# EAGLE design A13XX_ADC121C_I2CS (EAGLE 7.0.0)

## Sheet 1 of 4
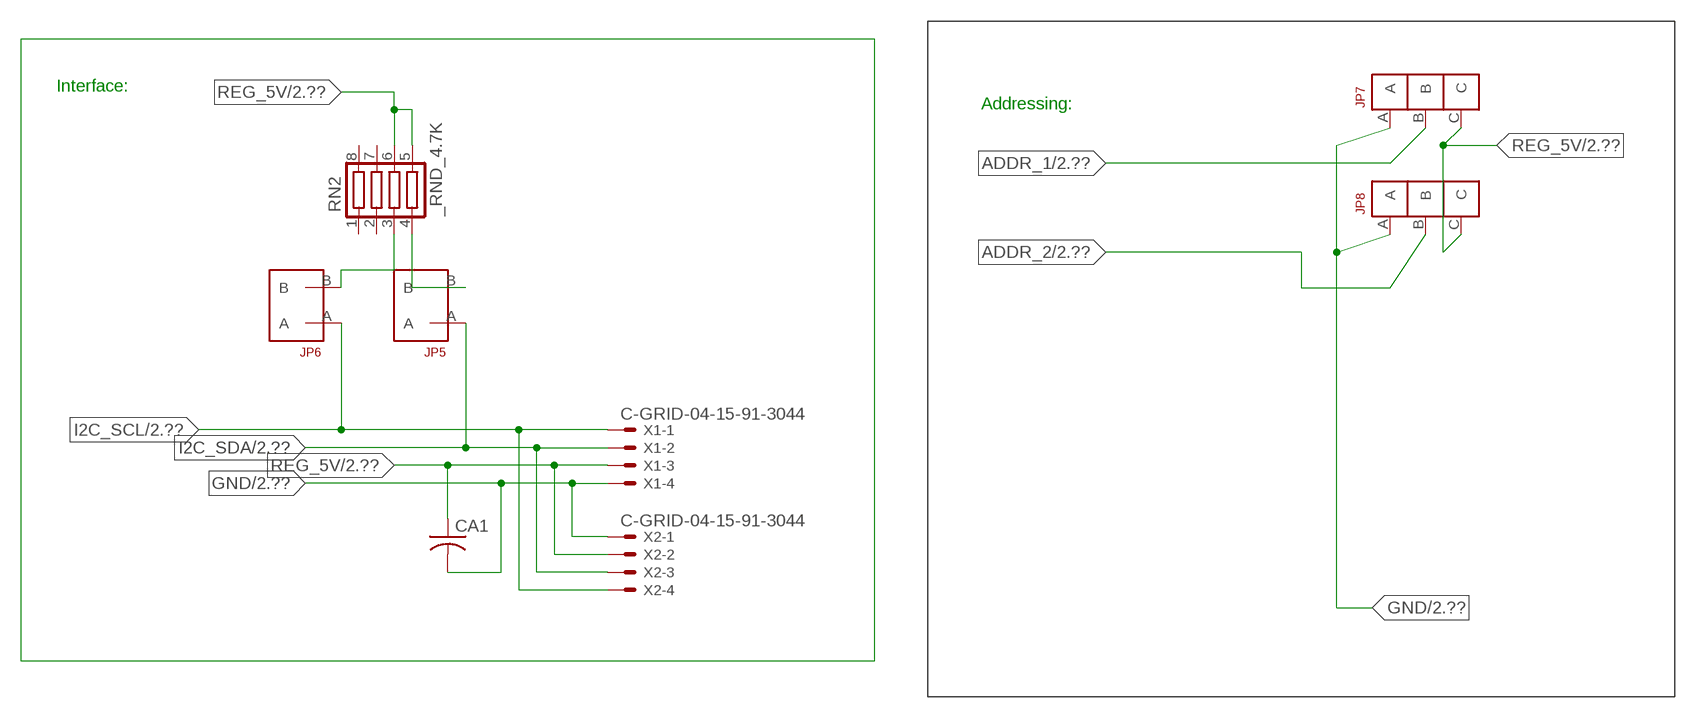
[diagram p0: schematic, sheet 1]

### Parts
CA1  CC1206KRX7R9BB104  [.1UF]
JP5  JUMPER_1X2_2MM  [JUMPER_1X2_2MM]
JP6  JUMPER_1X2_2MM  [JUMPER_1X2_2MM]
JP7  JUMPER_1X3_2MM  [JUMPER_1X3_2MM]
JP8  JUMPER_1X3_2MM  [JUMPER_1X3_2MM]
RN2  _RND_4.7K  [RND]
X1  C-GRID-04-15-91-3044  [15-91-04]
X2  C-GRID-04-15-91-3044  [15-91-04]

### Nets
ADDR_1: JP7.B ; also sheet 2
ADDR_2: JP8.B ; also sheet 2
GND: CA1.2 JP7.A JP8.A X1.4 X2.1 ; also sheet 2,3,4
I2C_SCL: JP6.A X1.1 X2.4 ; also sheet 2
I2C_SDA: JP5.A X1.2 X2.3 ; also sheet 2
N$1: JP6.B RN2.3
N$2: JP5.B RN2.4
REG_5V: CA1.1 JP7.C JP8.C RN2.5 RN2.6 X1.3 X2.2 ; also sheet 2,3,4
Unconnected: RN2.1 RN2.2 RN2.7 RN2.8

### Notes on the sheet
- Interface:
- Addressing:

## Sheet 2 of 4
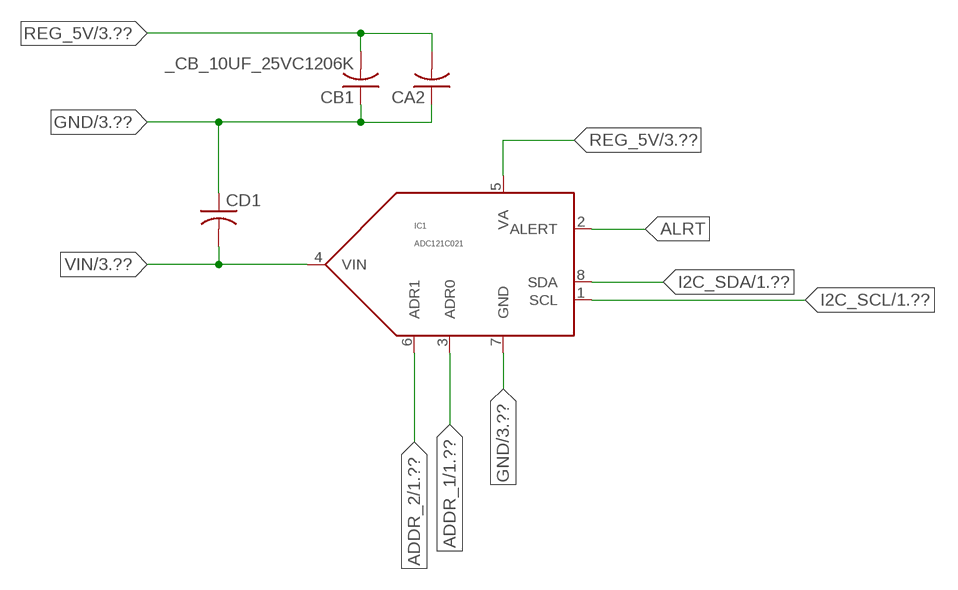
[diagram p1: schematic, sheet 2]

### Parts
CA2  _CA_.10UF_50VC1206K  [_CA_.1UF_50V]
CB1  _CB_10UF_25VC1206K  [_CB_10UF_25V]
CD1  _CD_10NF_50VC1206K  [_CD_10NF_50V]
IC1  ADC121C021  [MSOP08]

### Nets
ADDR_1: IC1.3(ADR0) ; also sheet 1
ADDR_2: IC1.6(ADR1) ; also sheet 1
ALRT: IC1.2(ALERT)
GND: CA2.1 CB1.1 CD1.1 IC1.7(GND) ; also sheet 1,3,4
I2C_SCL: IC1.1(SCL) ; also sheet 1
I2C_SDA: IC1.8(SDA) ; also sheet 1
REG_5V: CA2.2 CB1.2 IC1.5(VA) ; also sheet 1,3,4
VIN: CD1.2 IC1.4(VIN) ; also sheet 3

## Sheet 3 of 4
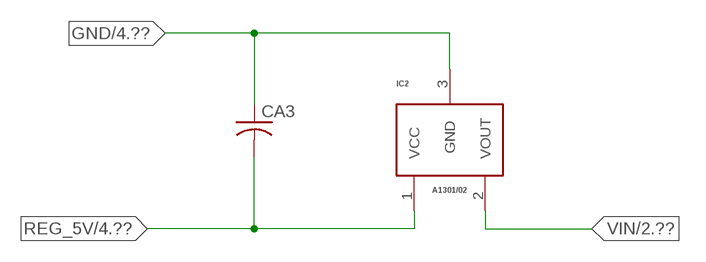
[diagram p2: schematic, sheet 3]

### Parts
CA3  _CA_.10UF_50VC1206K  [_CA_.1UF_50V]
IC2  A1301/02  [SOT23]

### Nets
GND: CA3.1 IC2.3(GND) ; also sheet 1,2,4
REG_5V: CA3.2 IC2.1(VCC) ; also sheet 1,2,4
VIN: IC2.2(VOUT) ; also sheet 2

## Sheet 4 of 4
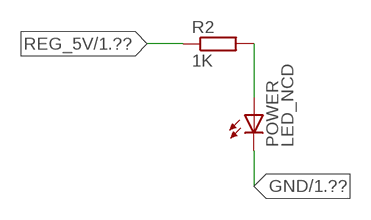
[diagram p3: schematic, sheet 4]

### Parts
POWER  LED_NCD  [CHIPLED_0603]
R2  1K  RESISTOR_SMT-0402  [R402]

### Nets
GND: POWER.C ; also sheet 1,2,3
N$13: POWER.A R2.2
REG_5V: R2.1 ; also sheet 1,2,3

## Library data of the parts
CA1 = NCD_ULTIMATE_LIBRARY:CC1206KRX7R9BB104: Capacitor CA .1uF 50V SMT C1206K CC1206KRX7R9BB104
CA2 CA3 = NCD_ULTIMATE_LIBRARY:_CA_.10UF_50V: Capacitor .1uF SMT
CB1 = NCD_ULTIMATE_LIBRARY:_CB_10UF_25V: Capacitor 10uF SMT
CD1 = NCD_ULTIMATE_LIBRARY:_CD_10NF_50V: Capacitor 10nF SMT
IC1 = NCD_ULTIMATE_bhaskar:ADC121C021: Digikey ADC121C021CIMM/NOPBCT-ND/ADC121C021CIMM/NOPB
IC2 = NCD_ULTIMATE_bhaskar:A1301/02: Digikey 620-1019-2-ND/A1301KLHLT-T 620-1021-2-ND/A1302KLHLT-T
JP5 JP6 = NCD_ULTIMATE_CONNECTORS:JUMPER_1X2_2MM
JP7 JP8 = NCD_ULTIMATE_CONNECTORS:JUMPER_1X3_2MM
POWER = NCD_ULTIMATE_LIBRARY:LED_NCD: LED Digikey 754-1132-2-ND/APT2012SRCPRV
R2 = NCD_ULTIMATE_LIBRARY:RESISTOR_SMT: NCD Resistor
RN2 = NCD_ULTIMATE_LIBRARY:_RND_4.7K: Resistor Array RND SMT 4.7K x 4 Single Resistor Source: http://www.ctscorp.com/components/Datasheets/CTSChipArrayDs.pdf Digikey 742C083472JPTR-ND/742C083472JP; OC_FARNELL: unknown; OC_NEWARK: unknown
X1 X2 = NCD_ULTIMATE_CONNECTORS:C-GRID-04: CONNECTOR 4-Pos I2C wire to board 2.54 mm (0.100") pitch header Digikey WM1342-ND/0015912045; OC_FARNELL: unknown; OC_NEWARK: unknown

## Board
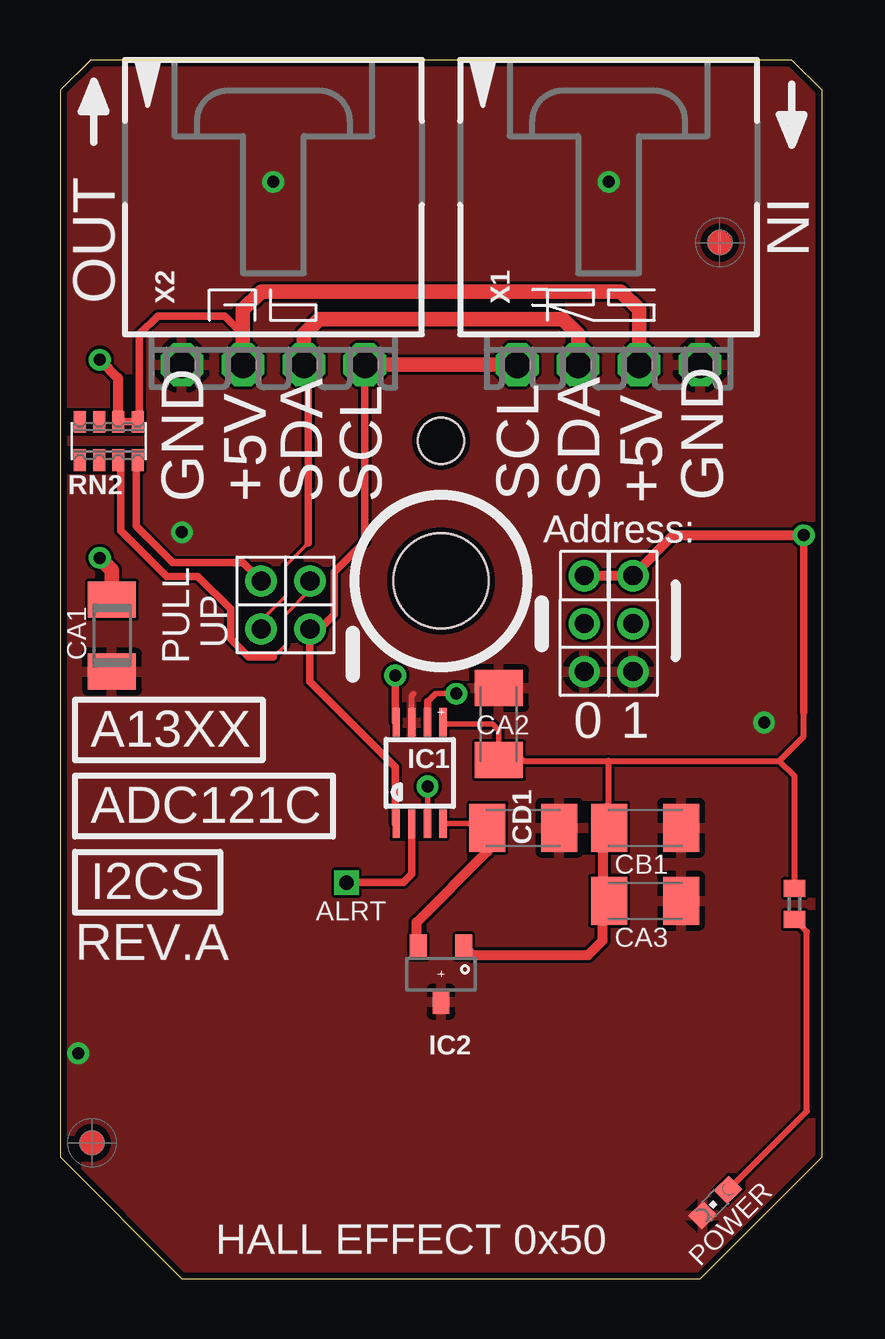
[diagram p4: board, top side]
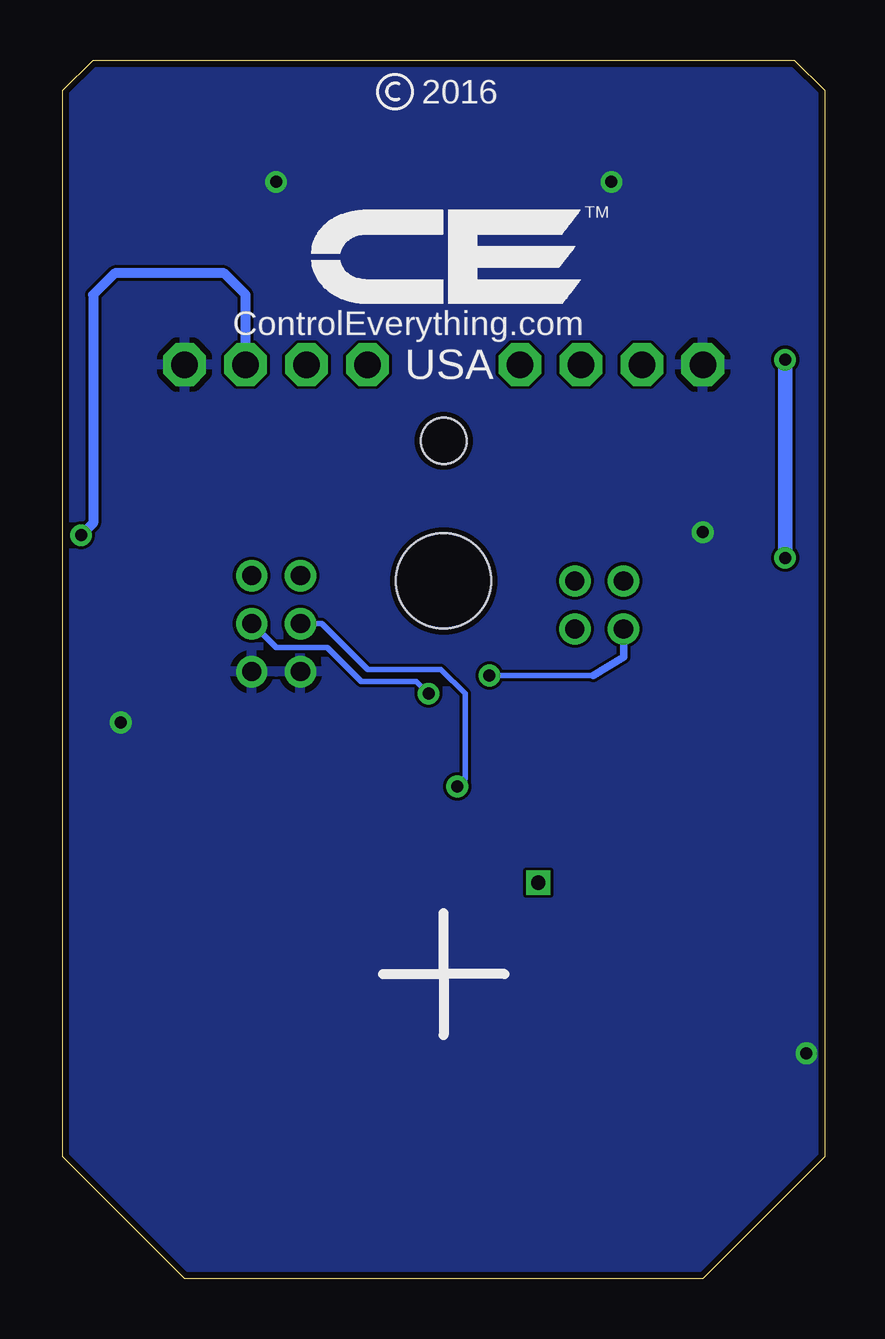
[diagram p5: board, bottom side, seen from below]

Size 31.75 x 50.8 mm. Coordinates in mm from the lower left corner, seen from the top.
Outline: 31.75,5.08 31.75,49.53 30.48,50.8 1.27,50.8 0,49.53 0,5.08 5.08,0 26.67,0 31.75,5.08
Outline: 31.75,5.08 31.75,49.53 30.48,50.8 1.27,50.8 0,49.53 0,5.08 5.08,0 26.67,0 31.75,5.08
Copper layers (1*16): Top 0.035mm / dielectric 1.5mm / Bottom 0.035mm
Design rules "default": minimum track width 5mil, minimum drill 24mil, track to track 5mil, track to pad 5mil, pad to pad 5mil, via to via 5mil, smd to smd 5mil, copper to edge 10mil, drill to drill 8mil, minimum pad ring 10mil, minimum via ring 8mil, stop-mask expansion 2mil, vias tented up to drill 0mil, thermal gap 10mil
Holes 3.96 mm at 15.88,29.08
Holes 1.91 mm at 15.88,34.92

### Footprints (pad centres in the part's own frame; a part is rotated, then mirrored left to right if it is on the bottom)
.1UF = smd 1.5 x 2: 1 -1.5,0; 2 1.5,0
_CA_.1UF_50V = smd 1.5 x 2: 1 -1.5,0; 2 1.5,0
_CB_10UF_25V = smd 1.5 x 2: 1 -1.5,0; 2 1.5,0
_CD_10NF_50V = smd 1.5 x 2: 1 -1.5,0; 2 1.5,0
MSOP08 = smd 0.3 x 1.2: 1 -0.976,-2.113; 2 -0.326,-2.113; 3 0.324,-2.113; 4 0.974,-2.113; 5 0.974,2.112; 6 0.324,2.112; 7 -0.326,2.112; 8 -0.976,2.112
SOT23 = smd 0.7 x 1: 1 -0.95,-1.15; 2 0.95,-1.15; 3 0,1.15
JUMPER_1X2_2MM = drill 0.8: A 0,2; B 0,0
JUMPER_1X3_2MM = drill 0.8: A 0,2; B 0,0; C 0,-2
CHIPLED_0603 = smd 0.8 x 0.876: A 0,-0.75; C 0,0.75
R402 = smd 0.7 x 0.9: 1 -0.65,0; 2 0.65,0
RND = smd 0.5 x 0.9: 1 -1.2,-0.8; 2 -0.4,-0.8; 3 0.4,-0.8; 4 1.2,-0.8; 5 1.2,0.8; 6 0.4,0.8; 7 -0.4,0.8; 8 -1.2,0.8
15-91-04 = drill 1.1 pad 1.778 octagon: 1 -3.81,-7.62; 2 -1.27,-7.62; 3 1.27,-7.62; 4 3.81,-7.62

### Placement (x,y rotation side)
CA1  2.16,26.81 270 top
CA2  18.29,23.11 270 top
CA3  24.38,15.75 180 top
CB1  24.38,18.8 180 top
CD1  19.3,18.8 180 top
IC1  14.99,21.08 0 top
IC2  15.88,12.7 180 top
JP5  8.38,29.08 180 top
JP6  10.41,29.08 180 top
JP7  21.84,27.31 180 top
JP8  23.88,27.31 180 top
POWER  27.3,3.18 135 top
R2  30.61,15.62 270 top
RN2  2.03,34.92 0 top
U$5  [VISION_REF10]  1.33,5.66 90 top
U$28  [VISION_REF10]  27.5,43.19 90 top
X1  22.86,45.72 0 top
X2  8.89,45.72 0 top

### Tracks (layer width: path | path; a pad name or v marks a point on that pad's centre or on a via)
ADDR_1  (via drill 0.5)
  Top 0.229: IC1.3 v15.32,20.52
  Bottom 0.229: v15.32,20.52 14.99,20.85 14.99,24.38 16,25.4 19.05,25.4 20.95,27.31 JP7.B 21.84,27.18
ADDR_2  (via drill 0.5)
  Top 0.229: 15.32,24.05 15.65,24.38 v16.51,24.38
  Top 0.305: IC1.6 15.32,24.05
  Bottom 0.229: v16.51,24.38 17.02,24.89 19.3,24.89 20.73,26.31 22.86,26.31 23.85,27.31 JP8.B
ALRT  (via drill 0.6)
  Top 0.305: IC1.2 14.66,16.87 14.3,16.51 v11.94,16.51
GND  (via drill 0.5)
  Top 0.254: IC1.7 14.66,24.31 14.73,24.38
  other vias: 8.89,45.72 22.86,45.72 29.34,23.19 0.76,9.4 5.08,31.12
  pour Top: -1.27,3.81 -1.27,50.8 0,52.07 31.75,52.07 33.02,50.8 33.02,3.81 27.94,-1.27 3.81,-1.27
  pour Bottom: 4.45,-0.63 -0.64,4.45 -0.64,50.17 0.64,51.44 31.11,51.44 32.38,50.17 32.38,4.45 27.3,-0.63
I2C_SCL
  Top 0.229: IC1.1 13.97,18.97
  Top 0.305: X2.4 12.7,30.73 11.43,29.46 11.43,27.69 10.83,27.08 JP6.A 10.41,24.89 13.97,21.34 13.97,18.97
  Top 0.61: X2.4 X1.1
I2C_SDA  (via drill 0.5)
  Top 0.152: 10.35,30.67 9.4,29.72 9.4,28.45 8.38,27.43 JP5.A
  Top 0.305: 10.35,30.67 10.35,37.91 X2.3 | IC1.8 13.97,23.23 v13.97,25.15
  Top 0.61: X2.3 10.16,39.37 10.79,40.01 20.95,40.01 21.59,39.37 X1.2
  Bottom 0.229: v13.97,25.15 9.65,25.15
  Bottom 0.305: 9.65,25.15 8.38,25.91 JP5.A
N$1
  Top 0.152: 8.89,25.91 9.4,26.42 9.4,27.69 10.41,28.7 JP6.B
  Top 0.305: RN2.3 2.54,34.02 2.54,31.18 4.45,29.27 5.75,29.27 7.11,27.91 7.11,26.67 7.87,25.91 8.89,25.91
N$2
  Top 0.305: RN2.4 3.17,34.07 3.17,31.37 4.7,29.85 6.1,29.85 6.35,29.85 7.62,29.85 JP5.B
N$13
  Top 0.254: POWER.A 31.11,6.99 31.11,14.46 R2.2
REG_5V  (via drill 0.5)
  Top 0.229: IC1.5 16.04,23.11 18.03,23.11 18.29,22.86 CA2.2 18.82,22.1 19.07,21.84 | 22.35,19.3 22.86,18.8 CB1.2 23.11,19.03
  Top 0.254: 19.07,21.84 19.33,21.59 22.86,21.59 | 22.86,21.59 29.97,21.59 | 29.97,21.59 30.99,22.61 30.99,23.62 | 22.35,19.3 22.86,19.81 22.86,21.59 | R2.1 30.61,20.96 29.97,21.59
  Top 0.305: 7.62,39.37 7.49,39.37 | RN2.6 RN2.5 3.3,35.8 3.3,39.37 4.06,40.13 6.86,40.13 7.62,39.37 | X2.2 7.62,39.37 | 30.99,23.62 v30.99,30.99
  Top 0.406: v1.65,38.3 2.41,37.54 2.41,35.74 RN2.6 | 22.86,18.8 22.61,18.54 22.61,15.24 | v21.84,29.21 21.94,29.31 JP8.C 25.56,30.99 v30.99,30.99 | IC2.1 17.19,13.49 22,13.49 22.61,14.1 22.61,15.24 | CA3.2 22.88,15.52 22.61,15.24
  Top 0.61: X1.3 24.13,38.23 24.13,40.39 23.37,41.15 8.38,41.15 7.62,40.39 X2.2 | CA1.1 2.16,29.54 v1.65,30.05
  Top 0.813: v30.99,30.99 31.05,30.99
  Bottom 0.229: JP7.C v21.84,29.21
  Bottom 0.406: X1.3 24.13,41.01 25.03,41.91 29.58,41.91 30.48,41.01 30.48,31.5 v30.99,30.99
  Bottom 0.61: v1.65,30.05 v1.65,38.3
VIN
  Top 0.229: IC1.4 17.55,18.97
  Top 0.305: 17.55,18.97 CD1.2 17.53,19.05
  Top 0.406: IC2.2 14.86,14.1 14.86,14.86 17.8,17.8 CD1.2

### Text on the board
tPlace: ALRT | HALL EFFECT 0x50
tNames: IN | OUT | GND | GND | +5V | +5V | SDA | SDA | SCL | SCL | SCL | SCL | SDA | SDA | +5V | +5V | GND | GND | Address: | Address: | PULL | UP | 0 | 1 | A13XX | ADC121C | I2CS | REV.A
bNames: 2016 | TM | ControlEverything.com | USA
